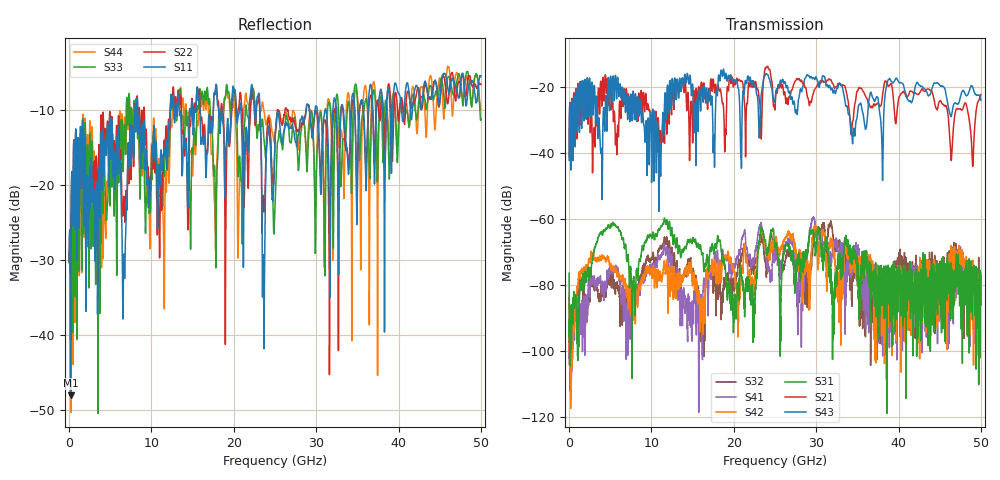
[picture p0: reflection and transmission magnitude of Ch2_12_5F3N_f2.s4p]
!Agilent Technologies,N5247A,US51170199,A.09.90.13
!Agilent N5247A: A.09.90.13
!Date: Tuesday, December 08, 2015 12:19:50
!Correction: S11(Full 4 Port(1,2,3,4))
!S12(Full 4 Port(1,2,3,4))
!S13(Full 4 Port(1,2,3,4))
!S14(Full 4 Port(1,2,3,4))
!S21(Full 4 Port(1,2,3,4))
!S22(Full 4 Port(1,2,3,4))
!S23(Full 4 Port(1,2,3,4))
!S24(Full 4 Port(1,2,3,4))
!S31(Full 4 Port(1,2,3,4))
!S32(Full 4 Port(1,2,3,4))
!S33(Full 4 Port(1,2,3,4))
!S34(Full 4 Port(1,2,3,4))
!S41(Full 4 Port(1,2,3,4))
!S42(Full 4 Port(1,2,3,4))
!S43(Full 4 Port(1,2,3,4))
!S44(Full 4 Port(1,2,3,4))
!S4P File: Measurements: <S11,S12,S13,S14>,
!<S21,S22,S23,S24>,
!<S31,S32,S33,S34>,
!<S41,S42,S43,S44>:
# Hz S  dB  R 50
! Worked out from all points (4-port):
!   3201 points, 10 MHz to 50 GHz, reference 50 ohm
!   strongest paths, dB at 10 MHz, 12.51 GHz, 25 GHz, 37.5 GHz, 50 GHz:
!     S43: -42.4, -17.9, -23.9, -23.6, -24.1
!     S21: -41.4, -21.6, -26.8, -25.0, -22.4
!     S31: -76.6, -63.6, -68.4, -81.9, -86.2
!     S42: -87.2, -76.3, -67.4, -74.9, -77.2
!     S41: -82.4, -73.5, -72.0, -84.3, -81.9
!     S32: -83.9, -69.6, -72.2, -83.7, -85.9
!   lowest |S11| = -48.0 dB at 181.8 MHz (marker M1), VSWR 1.01, Z = 50.1 - j0.385 ohm
!   |S11| at or under -10 dB: start of sweep to 7.974 GHz; 8.339 GHz to 12.28 GHz (3.945 GHz wide, 38.3 % of centre); 23.19 GHz to 28.8 GHz (5.604 GHz wide, 21.6 % of centre)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
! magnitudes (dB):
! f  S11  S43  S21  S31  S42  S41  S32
! 10 MHz  -30.2  -42.4  -41.4  -76.6  -87.2  -82.4  -83.9
! 181.8 MHz  -48.0  -29.6  -30.6  -100.6  -99.4  -103.0  -95.1
! 5.29 GHz  -16.4  -18.1  -23.0  -61.1  -74.5  -76.3  -77.3
! 11.04 GHz  -19.9  -38.2  -33.9  -63.2  -77.5  -71.9  -68.9
! 28.27 GHz  -10.7  -21.3  -18.4  -73.8  -76.9  -83.9  -73.3
! 29.66 GHz  -12.4  -17.3  -22.1  -64.4  -65.1  -59.8  -68.2
! 50 GHz  -5.4  -24.1  -22.4  -86.2  -77.2  -81.9  -85.9
